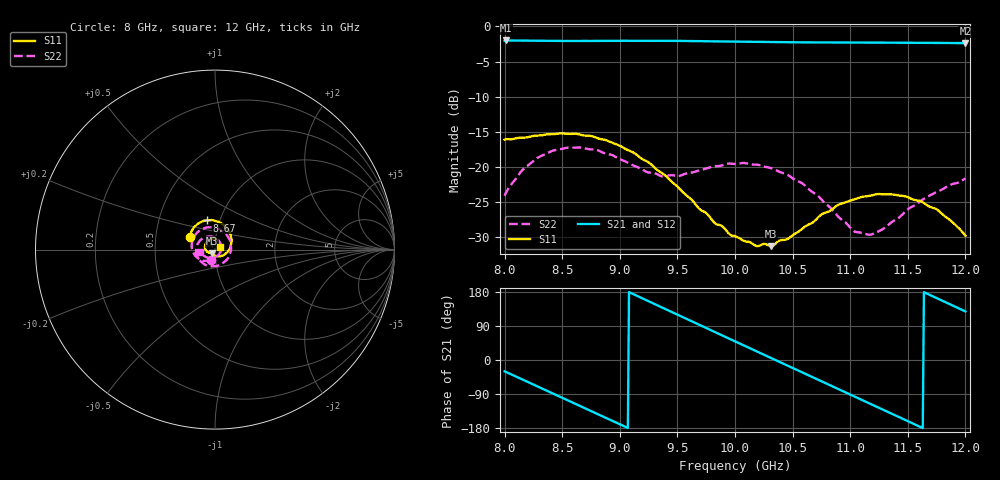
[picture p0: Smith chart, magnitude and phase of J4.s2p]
!Keysight Technologies,N5234A,MY52241180,A.10.60.03
!Date: Tuesday, May 30, 2023 15:21:05
!Correction: S11(Full 2 Port(1,2))
!S21(Full 2 Port(1,2))
!S12(Full 2 Port(1,2))
!S22(Full 2 Port(1,2))
!S2P File: Measurements: S11, S21, S12, S22:
# Hz S  dB  R 50
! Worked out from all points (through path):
!   401 points, 8 GHz to 12 GHz, reference 50 ohm
!   highest |S21| = -1.99 dB at 8.01 GHz (marker M1); lowest = -2.4 dB at 12 GHz (marker M2)
!   group delay of S21, straight-line fit = 390 ps
!   lowest |S11| = -31.3 dB at 10.31 GHz (marker M3), VSWR 1.06, Z = 48.2 - j1.94 ohm
!   |S11| at or under -10 dB: start of sweep to end of sweep
!   |S22| runs from -29.7 to -17.2 dB; largest |S21 - S12| = 0.0014
!   S11 on the Smith chart (normalised r, x): 8 GHz: 0.75, +0.11; 8.67 GHz: 0.87, +0.29; 12 GHz: 1.06, +0.03
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8e9  -16.13 153.9  -2.05 -29.9  -2.05 -29.9  -24.14 -110.4
8.01e9  -16.05 153.6  -1.99 -31.2  -2.00 -31.2  -23.76 -112.7
8.35e9  -15.42 135.4  -2.05 -78.8  -2.06 -78.8  -18.22 -173.4
8.51e9  -15.25 121.4  -2.06 -101.1  -2.07 -101.1  -17.39 160.4
8.67e9  -15.48 105.2  -2.06 -123.4  -2.07 -123.4  -17.26 133.2
8.85e9  -16.09 84.6  -2.05 -148.6  -2.06 -148.6  -17.96 101.4
9.01e9  -17.08 64.0  -2.04 -171.0  -2.05 -171.1  -18.99 70.1
9.17e9  -18.61 42.3  -2.03 166.4  -2.04 166.4  -20.16 33.5
9.34e9  -20.63 17.1  -2.03 142.3  -2.04 142.3  -21.20 -10.0
9.51e9  -22.99 -10.9  -2.05 118.2  -2.06 118.2  -21.33 -55.1
9.67e9  -25.64 -39.1  -2.09 95.6  -2.10 95.6  -20.61 -93.6
9.83e9  -28.09 -68.9  -2.12 73.1  -2.13 73.0  -19.91 -127.2
1e10  -29.87 -99.9  -2.17 49.2  -2.18 49.1  -19.61 -159.0
1.031e10  -31.32 -132.3  -2.23 5.8  -2.24 5.7  -20.19 150.2
1.049e10  -29.91 -142.6  -2.26 -19.4  -2.26 -19.5  -21.52 120.8
1.067e10  -27.99 -156.6  -2.27 -44.7  -2.28 -44.7  -23.57 90.3
1.084e10  -26.11 -172.7  -2.28 -68.5  -2.29 -68.5  -26.04 57.8
1.1e10  -24.81 167.8  -2.29 -91.0  -2.30 -91.0  -28.67 17.7
1.117e10  -24.15 144.8  -2.30 -114.9  -2.31 -114.9  -29.70 -34.1
1.134e10  -23.92 122.2  -2.31 -138.8  -2.32 -138.8  -28.15 -77.3
1.166e10  -25.40 74.5  -2.33 176.1  -2.34 176.1  -24.37 -132.4
1.2e10  -29.83 24.5  -2.37 128.2  -2.38 128.1  -21.69 -169.7
